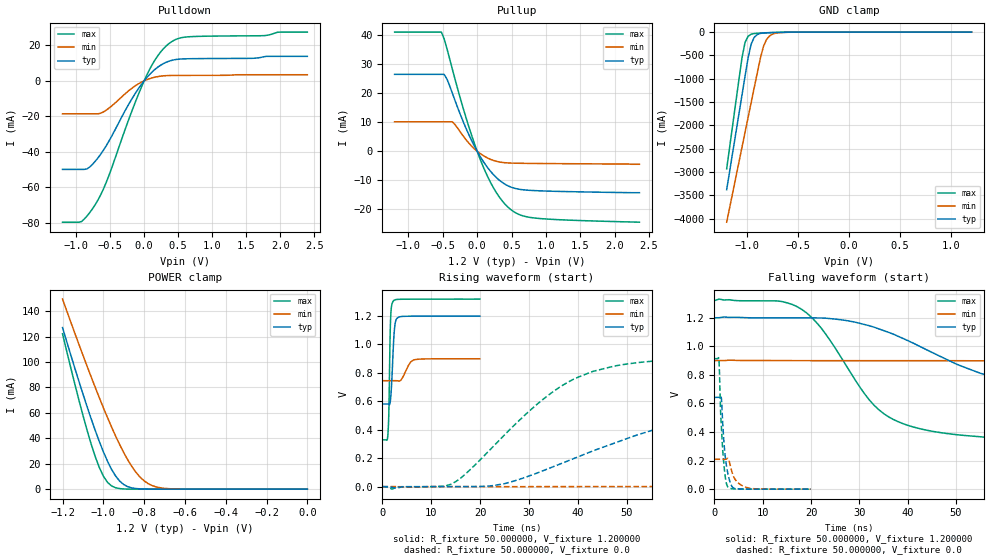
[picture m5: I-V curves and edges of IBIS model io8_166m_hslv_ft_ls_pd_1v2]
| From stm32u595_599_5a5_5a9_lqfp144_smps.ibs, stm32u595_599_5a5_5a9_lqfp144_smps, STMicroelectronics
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|   Model io8_166m_hslv_ft_ls_pd_1v2
[Model]  io8_166m_hslv_ft_ls_pd_1v2
Model_type I/O
Polarity   Non-Inverting
Enable   Active-Low
Vinl =   0.360000V
Vinh =   0.840000V
Vmeas =  0.600000V
Cref =   50.000000pF
Rref =   100.000000M
Vref =   0.0V
C_comp   3.151600pF   3.087200pF   3.197800pF
[Temperature Range]   25.000000   0.140000k   -40.000000
[Pullup Reference]   1.200000V   0.900000V   1.320000V
[Pulldown Reference]   0.0V   0.0V   0.0V
[POWER Clamp Reference]   1.200000V   0.900000V   1.320000V
[GND Clamp Reference]   0.0V   0.0V   0.0V
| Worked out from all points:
|   slope of the pulldown table from 0 to 0.18 V, typ, clamps not added: 25.4 ohm
|   slope of the pullup table from 0 to 0.18 V, typ, clamps not added: 27.8 ohm
|   GND clamp passes 1 mA (typ) near -0.51 V on its own axis
|   POWER clamp passes 1 mA (typ) near -0.86 V on its own axis
|   rising waveform, R_fixture 50.000000, V_fixture 1.200000: 20-80 % time 537ps typ, 1.37ns min, 302ps max; typ from 0.581 V to 1.2 V
|   rising waveform, R_fixture 50.000000, V_fixture 0.0: 20-80 % time 35.4ns typ, 88.4ns min, 17.9ns max; typ from 0 V to 0.642 V
|   falling waveform, R_fixture 50.000000, V_fixture 1.200000: 20-80 % time 31.1ns typ, 74.2ns min, 12.9ns max; typ from 1.2 V to 0.581 V
|   falling waveform, R_fixture 50.000000, V_fixture 0.0: 20-80 % time 1.03ns typ, 1.72ns min, 818ps max; typ from 0.642 V to 0 V
[Pulldown]
|Voltage   I(typ)   I(min)   I(max)
-1.2V     -49.86mA   -18.56mA   -79.56mA
-920mV    -49.86mA   -18.56mA   -79.19mA
-840mV    -49.6mA    -18.56mA   -76.08mA
-720mV    -45.32mA   -18.56mA   -69.74mA
-560mV    -36.71mA   -16.58mA   -57.44mA
-200mV    -11.43mA   -4.738mA   -19.03mA
0V        -10fA      -1.1pA     0A
160mV     6.477mA    2.074mA    11.78mA
360mV     10.99mA    2.988mA    20.81mA
480mV     12.07mA    3.052mA    23.53mA
640mV     12.43mA    3.072mA    24.76mA
2.4V      13.79mA    3.432mA    27.44mA
[Pullup]
|Voltage   I(typ)   I(min)   I(max)
-1.2V     26.49mA    10.13mA    41.07mA
-520mV    26.49mA    10.13mA    41.07mA
-480mV    26.49mA    10.13mA    38.77mA
-440mV    24.94mA    10.13mA    35.49mA
-360mV    19.99mA    10.13mA    28.26mA
-160mV    7.809mA    3.929mA    11.44mA
40mV      -1.648mA   -721uA     -2.521mA
240mV     -8.14mA    -3.199mA   -12.72mA
480mV     -12.27mA   -4.076mA   -19.94mA
640mV     -13.22mA   -4.166mA   -22.09mA
880mV     -13.63mA   -4.229mA   -23.14mA
2.36V     -14.3mA    -4.5mA     -24.47mA
[GND_clamp]
|Voltage   I(typ)   I(min)   I(max)
-1.2V     -3.379A    -4.076A    -2.932A
-1.05V    -1.35A     -2.47A     -550.7mA
-1.02V    -947.8mA   -2.15A     -221.5mA
-990mV    -552.4mA   -1.829A    -88.45mA
-960mV    -255.3mA   -1.51A     -44.89mA
-930mV    -111.8mA   -1.191A    -30.7mA
-870mV    -28.37mA   -564.6mA   -21.36mA
-840mV    -18.66mA   -309.5mA   -18.51mA
-810mV    -14.08mA   -161.6mA   -15.94mA
-780mV    -11.38mA   -83.33mA   -13.55mA
-600mV    -3.02mA    -4.329mA   -3.104mA
1.2V      30.28uA    18.17uA    37.27uA
[POWER_clamp]
|Voltage   I(typ)   I(min)   I(max)
-1.2V     127mA      149.4mA    122.2mA
-1.12V    84.97mA    114mA      70.27mA
-1.06V    55.51mA    88.42mA    35.67mA
-1.02V    37.63mA    72.04mA    17.17mA
-1V       29.51mA    64.13mA    10.3mA
-960mV    15.69mA    48.99mA    2.571mA
-900mV    3.624mA    28.77mA    182.8uA
-840mV    490.7uA    13.24mA    11.35uA
-800mV    116.8uA    6.532mA    1.77uA
-740mV    13.2uA     1.723mA    109.1nA
-620mV    167.4nA    79.36uA    0A
0V        0A         17.87nA    0A
[Ramp]
| variable   typ   min   max
dV/dt_r  0.38524/35.33371n   0.12523/88.29883n   0.54787/17.88662n
dV/dt_f  0.37097/31.06424n   92.56800m/74.12134n 0.59419/12.84584n
R_load = 50.000000
[Rising Waveform]
R_fixture= 50.000000
V_fixture= 1.200000
V_fixture_min= 0.900000
V_fixture_max= 1.320000
|time   V(typ)   V(min)   V(max)
0s        581.2mV    745.2mV    329.2mV
1.121ns   581.3mV    745.2mV    361.1mV
1.321ns   578.6mV    745.2mV    515mV
1.562ns   585.4mV    745.2mV    1.018V
1.682ns   618.2mV    745.2mV    1.176V
2.242ns   982.7mV    745.3mV    1.305V
2.643ns   1.153V     745.3mV    1.315V
3.403ns   1.193V     743mV      1.318V
6.406ns   1.199V     891.2mV    1.319V
19.94ns   1.2V       899.5mV    1.319V
[Rising Waveform]
R_fixture= 50.000000
V_fixture= 0.0
V_fixture_min= 0.0
V_fixture_max= 0.0
|time   V(typ)   V(min)   V(max)
0s        1.941nV    235.3nV    1.147nV
14.01ns   -237.5uV   -103.4uV   16.16mV
25.03ns   20.93mV    -77.03uV   365mV
38.04ns   182.2mV    99.47uV    736mV
48.05ns   313.3mV    341.3uV    851.8mV
60.06ns   442.8mV    1.614mV    893.3mV
82.08ns   573.8mV    19.78mV    909.9mV
115.1ns   629.7mV    76.35mV    912.9mV
235.2ns   642mV      194.8mV    913.1mV
498.5ns   642.1mV    208.9mV    913.1mV
[Falling Waveform]
R_fixture= 50.000000
V_fixture= 1.200000
V_fixture_min= 0.900000
V_fixture_max= 1.320000
|time   V(typ)   V(min)   V(max)
0s        1.2V       899.5mV    1.319V
17.02ns   1.198V     899.3mV    1.279V
22.02ns   1.198V     899.1mV    1.131V
31.03ns   1.152V     899.1mV    669.1mV
35.04ns   1.109V     899.1mV    528.4mV
43.04ns   989.9mV    899mV      419mV
57.06ns   791mV      897.6mV    361mV
82.08ns   652.1mV    878.9mV    335.7mV
127.1ns   593.2mV    805.6mV    329.4mV
498.5ns   581.2mV    745.2mV    329.2mV
[Falling Waveform]
R_fixture= 50.000000
V_fixture= 0.0
V_fixture_min= 0.0
V_fixture_max= 0.0
|time   V(typ)   V(min)   V(max)
0s        642.1mV    208.9mV    913.1mV
920.9ps   642.4mV    209mV      909.1mV
1.241ns   648.2mV    209.1mV    572.9mV
1.401ns   646mV      209.1mV    460.7mV
1.722ns   457.2mV    209.1mV    269.3mV
2.162ns   250.5mV    208.9mV    107.2mV
2.763ns   111.5mV    215.2mV    16.08mV
3.804ns   11.98mV    101.6mV    2.386mV
6.326ns   540.4uV    15.65mV    93.56uV
19.94ns   1.941nV    235.3nV    1.147nV
